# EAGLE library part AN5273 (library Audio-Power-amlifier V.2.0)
The AN5273 is a monolithic integrated circuit designed for 4.0 W (18 V, 8 W) output audio power amplifier. It is a dual channel SEPP IC suitable for stereo operation in TV application.
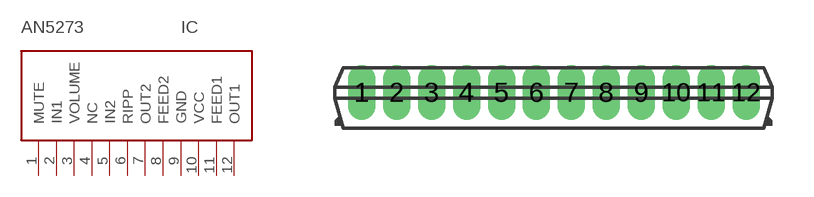
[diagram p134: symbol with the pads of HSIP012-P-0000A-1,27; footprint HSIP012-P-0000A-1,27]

Designator prefix IC

## AN5273  [HSIP012-P-0000A-1,27]
1  MUTE  in
2  IN1  in
3  VOLUME  in
4  NC  nc
5  IN2  in
6  RIPP
7  OUT2  out
8  FEED2
9  GND  pwr
10  VCC  pwr
11  FEED1
12  OUT1  out

## Footprint HSIP012-P-0000A-1,27 (pad centres in mm)
drill 0.5 long: 1 -7.62,0; 2 -6.35,0; 3 -5.08,0; 4 -3.81,0; 5 -2.54,0; 6 -1.27,0; 7 0,0; 8 1.27,0; 9 2.54,0; 10 3.81,0; 11 5.08,0; 12 6.35,0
